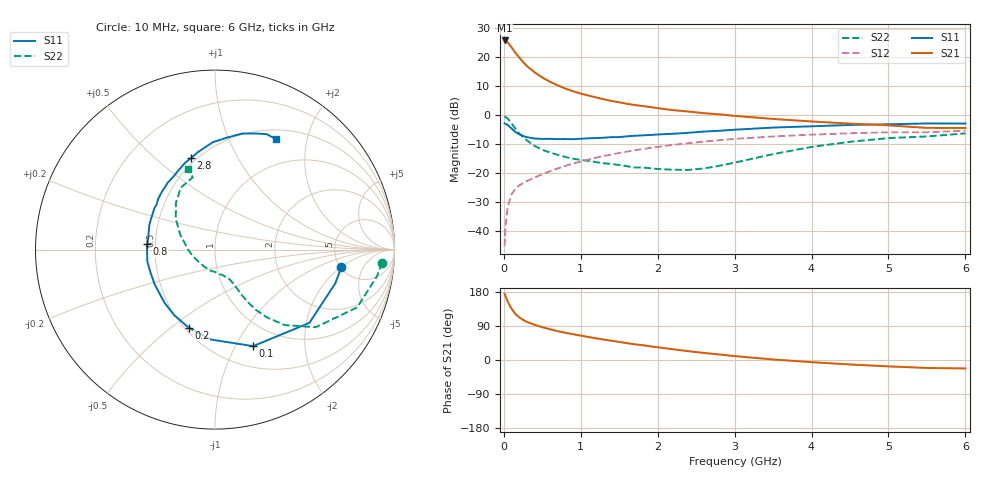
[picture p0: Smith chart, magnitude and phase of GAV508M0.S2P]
! Infineon Technologies  Discrete & RF Semiconductors
! BF775
! Si NPN RF Bipolar Junction Transistor in SOT23
! VCE = 0.5 V  IC = 8 mA
! Common Emitter S-Parameters:  May  1996
# GHz  S  MA  R  50
!  f  S11  S21  S12  S22
! GHz  MAG  ANG  MAG  ANG  MAG  ANG  MAG  ANG
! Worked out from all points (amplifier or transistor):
!   36 points, 10 MHz to 6 GHz, reference 50 ohm
!   highest |S21| = 25.6 dB at 10 MHz (marker M1)
!   |S21| within 3 dB of that: start of sweep to 117.4 MHz
!   unconditionally stable (mu >= 1): 409.6 MHz to end of sweep
!   at 250 MHz: K = 0.74, MSG = 20.9 dB, |S12| = -23.6 dB
!   at 1.4 GHz: K = 1.28, MAG = 6.0 dB, |S12| = -13.7 dB
!   at 6 GHz: K = 1.10, MAG = -1.5 dB, |S12| = -5.5 dB
!   S11 on the Smith chart (normalised r, x): 10 MHz: 5.08, -2.03; 100 MHz: 0.73, -1.18; 200 MHz: 0.52, -0.58; 800 MHz: 0.45, +0.03; 2.8 GHz: 0.47, +0.66; 6 GHz: 0.62, +1.51
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0.01  0.7109 -8.0  19.02 174.8  0.0054 84.2  0.9341 -4.5
0.02  0.696 -15.7  18.89 169.0  0.0112 83.0  0.9149 -9.3
0.05  0.6658 -37.8  17.64 154.4  0.0258 70.7  0.8552 -22.1
0.1  0.5785 -68.4  14.53 135.6  0.0425 59.8  0.7087 -37.6
0.15  0.5017 -92.6  11.68 121.5  0.0523 53.8  0.5735 -47.2
0.2  0.4589 -108.7  9.643 112.7  0.06 51.0  0.4771 -52.5
0.25  0.4297 -122.2  8.068 105.9  0.0661 50.0  0.4104 -55.6
0.3  0.4085 -133.5  6.893 100.5  0.0716 50.7  0.3594 -57.5
0.4  0.388 -150.0  5.359 92.8  0.0825 51.8  0.289 -59.7
0.5  0.3812 -160.5  4.368 86.6  0.0937 53.1  0.2474 -60.5
0.6  0.3829 -169.8  3.692 81.1  0.1061 54.1  0.223 -61.2
0.7  0.3786 -178.1  3.197 76.1  0.1179 54.8  0.2028 -62.4
0.8  0.3798 175.5  2.814 71.9  0.1306 55.1  0.1865 -63.7
1.1  0.3907 159.3  2.135 60.7  0.1683 54.3  0.1591 -69.7
1.3  0.4002 150.3  1.84 53.9  0.1936 52.9  0.1455 -74.9
1.6  0.4228 138.8  1.536 44.4  0.2305 49.9  0.129 -86.8
2.2  0.4682 119.6  1.196 28.3  0.3012 42.4  0.1122 -122.1
2.8  0.5271 104.6  1.013 14.6  0.363 34.0  0.1313 -166.4
3.5  0.5988 91.1  0.844 1.4  0.4203 23.6  0.2087 157.4
4.5  0.6639 76.8  0.701 -11.8  0.4776 10.1  0.3403 129.7
5.5  0.7047 65.9  0.591 -21.0  0.4972 -2.7  0.421 107.1
6  0.7029 61.3  0.589 -22.3  0.5288 -6.3  0.4754 108.5
